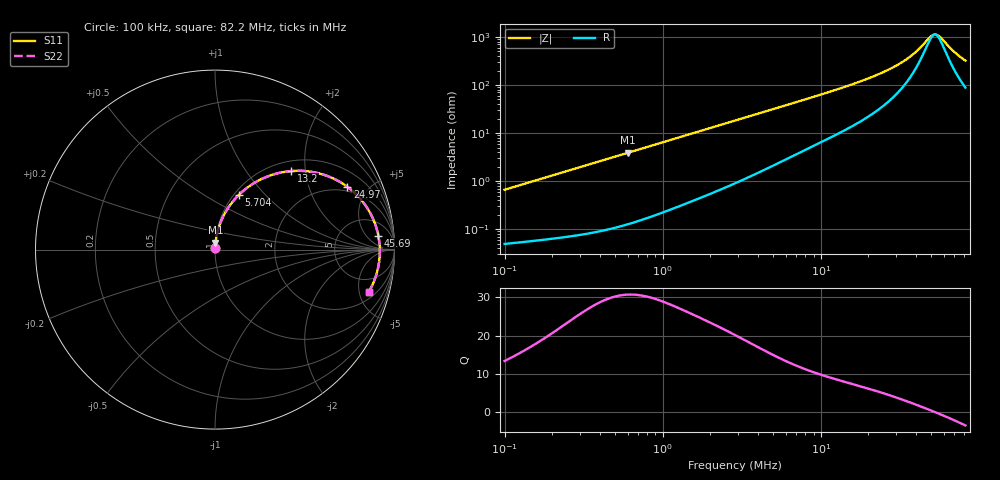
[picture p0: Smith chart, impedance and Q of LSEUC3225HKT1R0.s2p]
! LSEUC3225HKT1R0  S-PARAMETER MODEL  ( General Type )
! Model Generated by TAIYO YUDEN Corporation (http://www.ty-top.com)
! Version 1.0
! TAIYO YUDEN Control No. 211126
! Copyright(c) 2021 TAIYO YUDEN CO.,LTD. All Rights Reserved.
! Product Description (link to TY-COMPAS)
! https://ds.yuden.co.jp/TYCOMPAS/or/detail?pn=LSEUC3225HKT1R0M&u=M
! Products Name : Inductors
! Characteristics :
!  Inductance : 1.0 uH , SRF(min) : -Hz , DC Resistance(max) : 0.043 Ohm
!  Rated Current : Saturation :5200 mA , Temp Rise : 4200 mA (40 degC)
!  Case Size : 3.2 x 2.5 / 0.126 x 0.098 [mm/inch] , Thickness : 0.8 / 0.031 [mm/inch]
!  (Conditions: Temperature = 25 degC , DC Bias Current/Voltage = 0A / 0V)
! External Node Assignments :
!  1  o---GGG---o  2
! GND o---------o GND
! Frequency Range : 0.1MHz  -  82.198079MHz  [ 402 STEP ]
# MHz S RI R 50
! Freq[MHz].  S11 Real  S11 Imag  S21 Real  S21 Imag  S12 Real  S12 Imag  S22 Real  S22 Imag
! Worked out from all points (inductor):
!   401 points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, 100 kHz to 82.2 MHz, reference 50 ohm
!   read as one part in series: L = 1.05 uH near 103.4 kHz
!   highest Q = 30.8 at 602.2 kHz (marker M1), where L = 1.03 uH
!   self-resonance near 52.74 MHz
!   S11 on the Smith chart (normalised r, x): 100 kHz: 1.00, +0.01; 5.704 MHz: 1.05, +0.72; 13.2 MHz: 1.20, +1.68; 24.97 MHz: 1.74, +3.65; 45.69 MHz: 12, +11; 82.2 MHz: 2.77, -6.20
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0.1  0.000538 0.0066  0.9995 -0.0066  0.9995 -0.0066  0.000538 0.0066
0.307779  0.00117 0.02  0.9988 -0.02  0.9988 -0.02  0.00117 0.02
0.602179  0.00278 0.0388  0.9972 -0.0388  0.9972 -0.0388  0.00278 0.0388
0.947281  0.00576 0.0605  0.9942 -0.0605  0.9942 -0.0605  0.00576 0.0605
1.704233  0.0159 0.1066  0.9841 -0.1066  0.9841 -0.1066  0.0159 0.1066
2.867021  0.04 0.1728  0.96 -0.1728  0.96 -0.1728  0.04 0.1728
4.147136  0.0766 0.2377  0.9234 -0.2377  0.9234 -0.2377  0.0766 0.2377
5.704324  0.1313 0.3033  0.8687 -0.3033  0.8687 -0.3033  0.1313 0.3033
8.824095  0.2556 0.3914  0.7444 -0.3914  0.7444 -0.3914  0.2556 0.3914
13.19963  0.4256 0.4377  0.5744 -0.4377  0.5744 -0.4377  0.4256 0.4377
18.1559  0.5843 0.4234  0.4157 -0.4234  0.4157 -0.4234  0.5843 0.4234
24.97317  0.7372 0.35  0.2628 -0.35  0.2628 -0.35  0.7372 0.35
27.15873  0.7726 0.321  0.2274 -0.321  0.2274 -0.321  0.7726 0.321
31.58594  0.8282 0.2603  0.1718 -0.2603  0.1718 -0.2603  0.8282 0.2603
36.12361  0.8675 0.1984  0.1325 -0.1984  0.1325 -0.1984  0.8675 0.1984
40.62573  0.8932 0.1397  0.1068 -0.1397  0.1068 -0.1397  0.8932 0.1397
45.68896  0.9101 0.0779  0.0899 -0.0779  0.0899 -0.0779  0.9101 0.0779
50.52824  0.9174 0.0234  0.0826 -0.0234  0.0826 -0.0234  0.9174 0.0234
54.03595  0.9185 -0.0133  0.0815 0.0133  0.0815 0.0133  0.9185 -0.0133
57.78717  0.9166 -0.0501  0.0834 0.0501  0.0834 0.0501  0.9166 -0.0501
70.67687  0.8925 -0.1587  0.1075 0.1587  0.1075 0.1587  0.8925 -0.1587
82.19808  0.8568 -0.2356  0.1432 0.2356  0.1432 0.2356  0.8568 -0.2356
